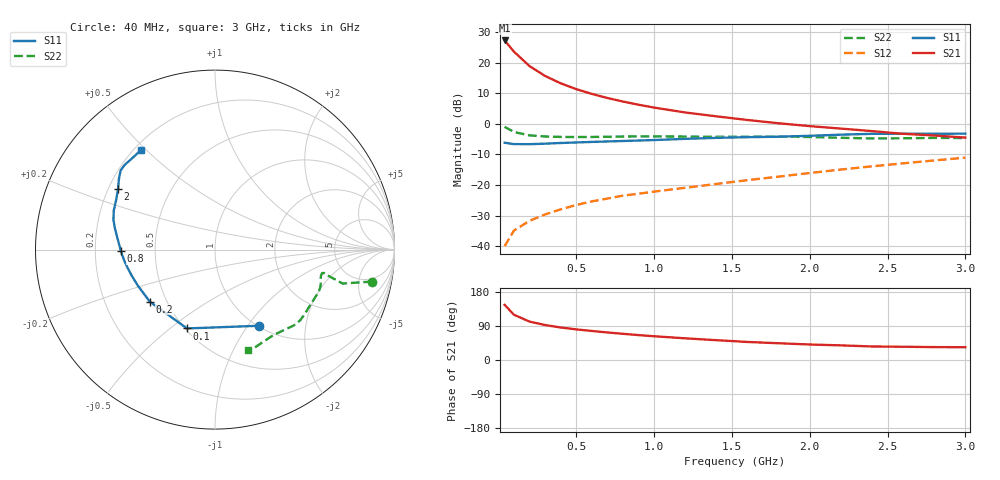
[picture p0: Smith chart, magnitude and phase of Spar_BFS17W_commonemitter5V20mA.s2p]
! Filename:  BFS17WE.S2P  Version:  4.0
! NXP part #: BFS17W  Date: Jun 1994
! Bias condition: Vce=5V, Ic=20mA
#  MHz  S  MA  R  50
! Freq  S11  S21  S12  S22  !GUM [dB]
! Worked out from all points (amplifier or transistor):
!   21 points, 40 MHz to 3 GHz, reference 50 ohm
!   highest |S21| = 27.3 dB at 40 MHz (marker M1)
!   |S21| within 3 dB of that: start of sweep to 89.22 MHz
!   unconditionally stable (mu >= 1): 264.4 MHz to 2.078 GHz
!   at 300 MHz: K = 1.06, MAG = 21.1 dB, |S12| = -29.6 dB
!   at 1 GHz: K = 1.24, MAG = 10.8 dB, |S12| = -22.2 dB
!   at 3 GHz: K = 0.97, MSG = 3.3 dB, |S12| = -11.1 dB
!   S11 on the Smith chart (normalised r, x): 40 MHz: 1.02, -1.14; 100 MHz: 0.51, -0.57; 200 MHz: 0.40, -0.30; 800 MHz: 0.31, -0.01; 2 GHz: 0.24, +0.27; 3 GHz: 0.23, +0.48
40  0.491 -59.8  23.06 145.6  0.01 69.3  0.893 -11.5
100  0.466 -109.5  15.14 119.4  0.018 58.7  0.736 -14.9
200  0.465 -141.4  8.783 101.4  0.026 59.6  0.648 -13.0
300  0.474 -154.7  6.06 92.3  0.033 62.1  0.621 -12.1
400  0.486 -162.5  4.599 85.8  0.04 65.0  0.611 -12.4
500  0.496 -167.6  3.689 80.8  0.047 67.1  0.608 -13.6
600  0.506 -171.8  3.085 76.6  0.054 69.0  0.61 -15.1
700  0.515 -175.5  2.646 72.7  0.06 70.5  0.614 -16.6
800  0.524 -179.0  2.315 69.1  0.067 71.9  0.62 -18.2
900  0.533 177.6  2.054 65.7  0.072 73.5  0.623 -19.7
1000  0.543 174.4  1.843 62.7  0.078 75.2  0.624 -21.3
1200  0.568 168.5  1.533 57.2  0.09 78.7  0.619 -25.1
1400  0.59 163.6  1.326 52.3  0.104 82.3  0.614 -30.0
1600  0.605 158.7  1.155 47.6  0.12 85.0  0.615 -35.2
1800  0.616 153.4  1.022 44.2  0.137 87.8  0.617 -39.7
2000  0.637 148.0  0.917 40.9  0.157 89.8  0.609 -44.0
2200  0.665 143.6  0.836 38.6  0.179 91.1  0.591 -49.2
2400  0.686 140.1  0.76 35.7  0.202 91.8  0.577 -55.8
2600  0.69 136.8  0.687 35.0  0.226 91.6  0.58 -62.6
2800  0.687 132.1  0.645 34.0  0.252 91.3  0.589 -67.9
3000  0.691 126.7  0.595 33.8  0.28 90.8  0.586 -72.0
